PROGRAM MAIN
VAR CONSTANT
    cInitSource			: ST_MA_MultiArray_InitPars 
							:= ( eTypeCode := eMA_TypeCode_LREAL, nDims := 2, aDimSizes := [cChannels, cBufferLength]);
	
END_VAR

VAR
	(* Input *)	
	nInputSelection			: UDINT := 1;						// Switch between hardware and function generator	
	nSample					: UDINT;
	// Hardware
	aEl3632Ch1 AT %I*		: ARRAY[1..cOversamples] OF INT;	// Input from hardware e.g. EL3632 ch1
	aEl3632Ch2 AT %I*		: ARRAY[1..cOversamples] OF INT;	// Input from hardware e.g. EL3632 ch2
	// Function generator
	fbFunctionGenerator1	: FB_FunctionGenerator;		// Signal Generator, ch1
	fSetFrequency1			: LREAL := 400;		        // Hz
	fSetAmplitude1			: LREAL := 4;		        // peak amplitude of sin signal [m/s^2]
	fbFunctionGenerator2	: FB_FunctionGenerator;		// Signal Generator, ch2
	fSetFrequency2			: LREAL := 35;		        // Hz
	fSetAmplitude2			: LREAL := 4;		        // peak amplitude of sin signal	[m/s^2]	
		
	
	(* Input from aBuffer to fbSource *)
	aBuffer				: ARRAY[1..cChannels] OF ARRAY[1..cOversamples] OF LREAL;						
	fbSource			: FB_CMA_Source :=(	stInitPars := cInitSource, 
											nOwnID := eID_Source, 
											aDestIDs := [eID_IntRMS]);		// Initialize source buffers
										
	(* From fbSink to aRMSResult *)	
	aRMSResult   		: ARRAY[1..cChannels] OF ARRAY[1..cResult_Length] OF LREAL;	// Copy result									
	fbSink				: FB_CMA_Sink := (nOwnID := eID_Sink);

	
	(* Classify calculated RMS values *)
	nCountResults		  : ULINT;	
	bCalculate			  : BOOL;
	nChannel              : UDINT;
	ISOClassIs_Vel        : ARRAY[1..cChannels] OF E_IsoClass;
	ISOClassIs_Displ      : ARRAY[1..cChannels] OF E_IsoClass;	
	
	(* error monitoring *)
	fbErrHist			: FB_HRErrHist; 

	(* little helper variables *)
	Ch1VelRMS : LREAL;
	Ch1DisplRMS : LREAL;
	Ch2VelRMS : LREAL;
	Ch2DisplRMS : LREAL;	
	
	(* output *)
	ISO_10816_Classification AT%Q* : E_IsoClass;
	
END_VAR

(* Input *)
CASE nInputSelection OF
	0:  (* input from EL3632 *)
		FOR nSample := 1 TO cOversamples DO
			aBuffer[1][nSample] := cScale*INT_TO_LREAL(aEl3632Ch1[nSample]); // convert from Volts to acceleration in m/s^2
			aBuffer[2][nSample] := cScale*INT_TO_LREAL(aEl3632Ch2[nSample]);
		END_FOR 
	1:  (* signal generator *)		
		fbFunctionGenerator1(	fFrequency 	:= fSetFrequency1,
								fAmplitude 	:= fSetAmplitude1,
								eFunction 	:= E_FunctionType.Sine,
								aSignal		:= aBuffer[1] );	
		fbFunctionGenerator2(	fFrequency 	:= fSetFrequency2,
								fAmplitude 	:= fSetAmplitude2,
								eFunction 	:= E_FunctionType.Sine,
								aSignal		:= aBuffer[2] );	
END_CASE					

(* Call source to collect data *)
fbSource.Input2D( pDataIn 			:= ADR(aBuffer),
				  nDataInSize 		:= SIZEOF(aBuffer), 
				  eElementType 		:= eMA_TypeCode_LREAL,
				  nWorkDim0			:= 0,
				  nWorkDim1			:= 1,
				  pStartIndex		:= 0,
				  nOptionPars		:= cCMA_Option_MarkInterruption ); 
IF fbSource.bError THEN
	fbErrHist.AddError(bErr:=TRUE, hrErrCode:=fbSource.hrErrorCode, sErrSource:='MAIN.fbSource'); // error monitoring
	// ToDo: if error
END_IF

(* Push results to sink *)
fbSink.Output2D(	pDataOut 		:= ADR(aRMSResult), 
					nDataOutSize 	:= SIZEOF(aRMSResult), 
					eElementType 	:= eMA_TypeCode_LREAL, 
					nWorkDim0 		:= 0,
					nWorkDim1 		:= 1,
					nElementsDim0	:= 0,
					nElementsDim1	:= 0,
					pStartIndex 	:= 0,
					nOptionPars		:= 0,
					bNewResult		=> bCalculate );
IF fbSink.bError THEN
	fbErrHist.AddError(bErr:=TRUE, hrErrCode:=fbSink.hrErrorCode, sErrSource:='MAIN.fbSink'); // error monitoring
	// ToDo: if error
END_IF

// define class according to ISO 10816-3 based on velocity and displacement data for each measurement channel
IF bCalculate THEN
	Ch1VelRMS := aRMSResult[1][2];
	Ch1DisplRMS := aRMSResult[1][3];
	Ch2VelRMS := aRMSResult[2][2];
	Ch2DisplRMS := aRMSResult[2][3];	
	
	IF NOT lrealisnan(Ch1VelRMS) THEN 

		nCountResults := fbSink.nCntResults;
		
		// do for each channel
		FOR nChannel := 1 TO cChannels DO
			
			// evaluate velocity data
			ISOClassIs_Vel[nChannel] := E_IsoClass.A;
			IF aRMSResult[nChannel][2] > cISOClassDef_Velocity[3] THEN
				ISOClassIs_Vel[nChannel] := E_IsoClass.D;
			ELSIF aRMSResult[nChannel][2] > cISOClassDef_Velocity[2] THEN
				ISOClassIs_Vel[nChannel] := E_IsoClass.C;
			ELSIF aRMSResult[nChannel][2] > cISOClassDef_Velocity[1] THEN
				ISOClassIs_Vel[nChannel] := E_IsoClass.B;
			END_IF;  
			
			// evaluate displacement data
			ISOClassIs_Displ[nChannel] := E_IsoClass.A;
			IF aRMSResult[nChannel][3] > cISOClassDef_Displ[3] THEN
				ISOClassIs_Displ[nChannel] := E_IsoClass.D;
			ELSIF aRMSResult[nChannel][3] > cISOClassDef_Displ[2] THEN
				ISOClassIs_Displ[nChannel] := E_IsoClass.C;
			ELSIF aRMSResult[nChannel][3] > cISOClassDef_Displ[1] THEN
				ISOClassIs_Displ[nChannel] := E_IsoClass.B;
			END_IF;	
									
		END_FOR;
		
		// according to ISO 10816-3 select worst case 		
		ISO_10816_Classification := E_IsoClass.A;
		FOR  nChannel := 1 TO cChannels DO 
			IF ISOClassIs_Vel[nChannel] >  ISO_10816_Classification THEN
				ISO_10816_Classification := ISOClassIs_Vel[nChannel];
			END_IF
			IF ISOClassIs_Displ[nChannel] >  ISO_10816_Classification THEN
				ISO_10816_Classification := ISOClassIs_Displ[nChannel];
			END_IF
		END_FOR;
	ELSE
		// result is NaN... code here what to do. 
		
	END_IF;
	
END_IF

END_PROGRAM
